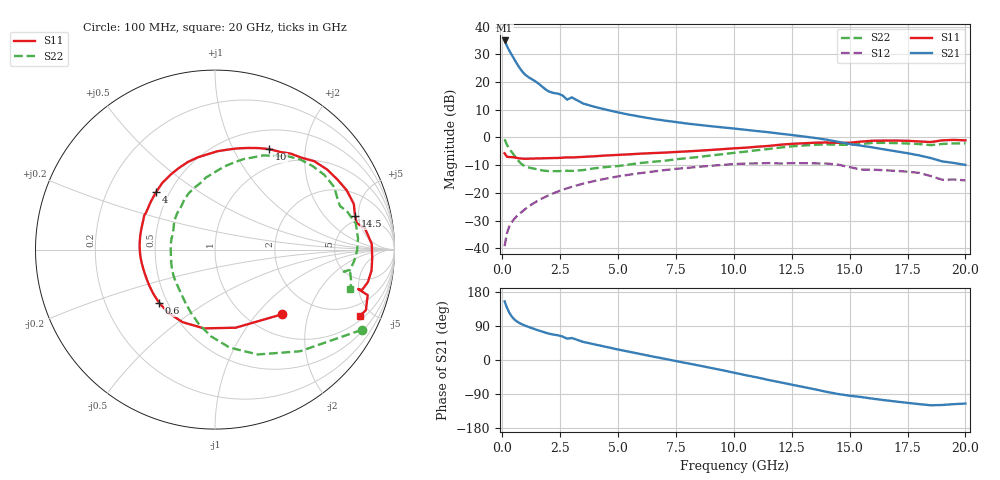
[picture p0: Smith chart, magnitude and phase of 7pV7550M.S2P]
! Infineon Technologies  Discrete & RF Semiconductors
! bfp620
! VCE = 0.75 V,  IC =  50 mA
! Common Emitter S-Parameters:  Sep 2002
# GHz  S  MA  R  50
!  f  S11  S21  S12  S22
! GHz  MAG  ANG  MAG  ANG  MAG  ANG  MAG  ANG
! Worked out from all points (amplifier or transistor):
!   59 points, 100 MHz to 20 GHz, reference 50 ohm
!   highest |S21| = 35.0 dB at 100 MHz (marker M1)
!   |S21| within 3 dB of that: start of sweep to 260.6 MHz
!   unconditionally stable (mu >= 1): 2.645 GHz to 2.932 GHz; 3.188 GHz to 10.35 GHz; 17 GHz to end of sweep
!   at 1 GHz: K = 0.87, MSG = 24.2 dB, |S12| = -25.8 dB
!   at 5.5 GHz: K = 1.04, MAG = 9.5 dB, |S12| = -13.4 dB
!   at 20 GHz: K = 1.48, MAG = -1.3 dB, |S12| = -15.5 dB
!   S11 on the Smith chart (normalised r, x): 100 MHz: 1.39, -1.37; 600 MHz: 0.45, -0.33; 4 GHz: 0.42, +0.34; 10 GHz: 0.74, +1.40; 14.5 GHz: 4.27, +4.49; 20 GHz: 1.23, -4.27
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0.1  0.518 -44.2  56.54 154.6  0.0109 75.3  0.9315 -28.7
0.2  0.4501 -75.2  44.75 138.3  0.0187 63.9  0.7384 -50.1
0.3  0.4432 -98.0  37.23 125.1  0.0247 60.1  0.631 -67.8
0.4  0.4428 -114.1  31.52 115.4  0.0293 58.4  0.5521 -81.5
0.5  0.4377 -126.5  26.73 108.3  0.0333 57.6  0.4839 -92.6
0.6  0.4299 -136.5  22.68 103.0  0.0369 57.3  0.4249 -102.2
0.8  0.4173 -151.7  16.81 95.7  0.0439 57.3  0.3415 -118.4
1  0.4134 -161.7  13.54 90.4  0.0513 57.4  0.3007 -130.9
1.4  0.4171 -174.5  10.52 81.5  0.0668 56.6  0.2724 -148.3
1.8  0.4215 174.2  7.804 73.4  0.0823 54.5  0.2523 -165.6
2  0.4237 169.3  6.808 69.8  0.09 53.1  0.2475 -173.1
2.8  0.4376 154.2  4.823 56.2  0.1209 46.4  0.2507 165.2
3  0.4359 151.9  5.299 58.1  0.1286 44.6  0.2488 164.9
3.5  0.4464 143.2  4.094 47.7  0.1472 39.6  0.2582 153.6
4  0.4586 135.9  3.566 41.0  0.1645 34.5  0.2783 144.7
7  0.5329 94.3  2.024 3.4  0.2573 3.4  0.3793 102.5
10  0.6367 61.6  1.453 -33.4  0.3313 -30.3  0.5281 72.6
10.5  0.6538 56.3  1.378 -39.9  0.3382 -37.0  0.5549 67.7
13.5  0.8049 24.2  0.982 -77.4  0.3407 -72.6  0.7377 34.3
14.5  0.8024 13.5  0.836 -89.7  0.3234 -87.7  0.7389 22.5
17  0.88 -7.6  0.564 -109.6  0.2495 -103.4  0.792 -0.3
20  0.8876 -24.5  0.32 -115.0  0.1681 -114.3  0.782 -16.4
